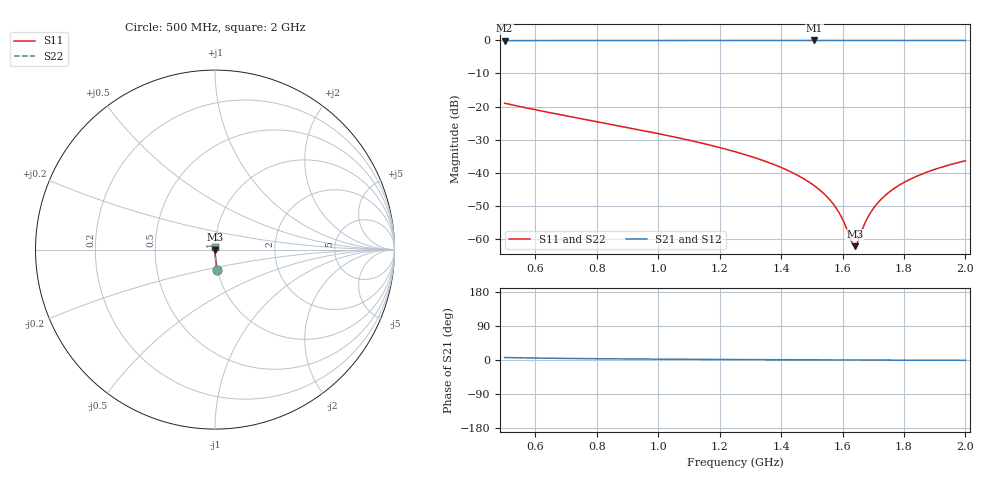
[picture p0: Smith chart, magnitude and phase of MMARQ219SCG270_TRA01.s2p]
! MMARQ219SCG270_TRA01  S-PARAMETER MODEL  ( General Type )
! Model Generated by TAIYO YUDEN Corporation (http://www.ty-top.com)
! Version 1.0
! TAIYO YUDEN Control No. 150609
! Copyright(c) 2015 TAIYO YUDEN CO.,LTD. All Rights Reserved.
! Product Description (link to TY-COMPAS)
! https://ds.yuden.co.jp/TYCOMPAS/or/detail?pn=MMARQ219SCG270JTRA01&u=M
! Products Name : Multilayer Ceramic Capacitors
! Characteristics :
!  Capacitance : 27 pF , Rated Voltage : 250V , TCC : CG / C0G
!  Case Size : 2.0 x 1.25 / 0.079 x 0.049 [mm/inch] , Thickness : 0.85 / 0.033 [mm/inch]
!  (Conditions: Temperature = 25 degC , DC Bias Current/Voltage = 0A / 0V)
! External Node Assignments :
!  1  o---| |---o  2
! GND o---------o GND
! Frequency Range : 500MHz  -  2GHz  [ 401 STEP ]
# MHz S RI R 50
! Freq[MHz].  S11 Real  S11 Imag  S21 Real  S21 Imag  S12 Real  S12 Imag  S22 Real  S22 Imag
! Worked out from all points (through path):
!   401 points, 500 MHz to 2 GHz, reference 50 ohm
!   highest |S21| = -0.01 dB at 1.509 GHz (marker M1); lowest = -0.1 dB at 500 MHz (marker M2)
!   group delay of S21, straight-line fit = 11.9 ps
!   lowest |S11| = -62.2 dB at 1.64 GHz (marker M3), VSWR 1.00, Z = 50.1 + j0.00343 ohm
!   |S11| at or under -10 dB: start of sweep to end of sweep
!   |S22| runs from -62.2 to -19.0 dB; largest |S21 - S12| = 0
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500  0.0129 -0.1115  0.9871 0.1115  0.9871 0.1115  0.0129 -0.1115
751.25  0.00469 -0.0651  0.9953 0.0651  0.9953 0.0651  0.00469 -0.0651
1002.5  0.00204 -0.0387  0.998 0.0387  0.998 0.0387  0.00204 -0.0387
1250  0.00107 -0.0207  0.9989 0.0207  0.9989 0.0207  0.00107 -0.0207
1396.25  0.000845 -0.0122  0.9992 0.0122  0.9992 0.0122  0.000845 -0.0122
1452.5  0.000799 -0.00916  0.9992 0.00916  0.9992 0.00916  0.000799 -0.00916
1501.25  0.000775 -0.00665  0.9992 0.00665  0.9992 0.00665  0.000775 -0.00665
1508.75  0.000773 -0.00627  0.9992 0.00627  0.9992 0.00627  0.000773 -0.00627
1546.25  0.000765 -0.00441  0.9992 0.00441  0.9992 0.00441  0.000765 -0.00441
1576.25  0.000763 -0.00296  0.9992 0.00296  0.9992 0.00296  0.000763 -0.00296
1602.5  0.000765 -0.00171  0.9992 0.00171  0.9992 0.00171  0.000765 -0.00171
1628.75  0.00077 -0.000485  0.9992 0.000485  0.9992 0.000485  0.00077 -0.000485
1640  0.000773 3.43e-05  0.9992 -3.43e-05  0.9992 -3.43e-05  0.000773 3.43e-05
1647.5  0.000775 0.000379  0.9992 -0.000379  0.9992 -0.000379  0.000775 0.000379
1673.75  0.000785 0.00157  0.9992 -0.00157  0.9992 -0.00157  0.000785 0.00157
1692.5  0.000793 0.00241  0.9992 -0.00241  0.9992 -0.00241  0.000793 0.00241
1718.75  0.000807 0.00357  0.9992 -0.00357  0.9992 -0.00357  0.000807 0.00357
1752.5  0.000829 0.00504  0.9992 -0.00504  0.9992 -0.00504  0.000829 0.00504
1797.5  0.000863 0.00696  0.9991 -0.00696  0.9991 -0.00696  0.000863 0.00696
1853.75  0.000915 0.0093  0.9991 -0.0093  0.9991 -0.0093  0.000915 0.0093
1925  0.000994 0.0122  0.999 -0.0122  0.999 -0.0122  0.000994 0.0122
2000  0.00109 0.0151  0.9989 -0.0151  0.9989 -0.0151  0.00109 0.0151
